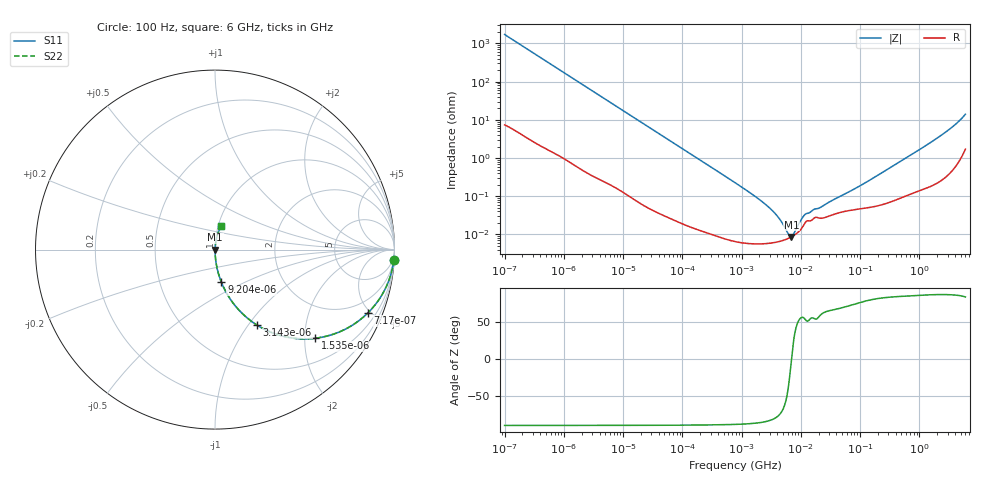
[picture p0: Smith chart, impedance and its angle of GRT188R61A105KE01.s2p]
!Murata Part Number: GRT188R61A105KE01
!These Parameters are Measured in Series Mode Connection
!Data Generated on Jun 19, 2026
!  o--ll--o
!Port1  Port2
!  o------o
!Operation Temp=25[degC], DC Bias Voltage=0[V]
!Freq. Start=100[Hz] Stop=6[GHz] 401[Steps]
# Hz S RI R 50
!Freq.(Hz) S11(Real) S11(Imag) S21(Real) S21(Imag) S12(Real) S12(Imag) S22(Real) S22(Imag)
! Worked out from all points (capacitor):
!   401 points, 100 Hz to 6 GHz, reference 50 ohm
!   read as one part in series: C = 928 nF near 109 Hz
!   lowest |Z| = 8.66 mohm at 6.949 MHz (marker M1)
!   series resonance near 6.96 MHz, so ESL is about 560 pH
!   S11 on the Smith chart (normalised r, x): 100 Hz: 1, -34; 717 Hz: 1.03, -4.81; 1.535 kHz: 1.01, -2.25; 3.143 kHz: 1.01, -1.10; 9.204 kHz: 1.00, -0.38; 6 GHz: 1.03, +0.28
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100  0.9964 -0.0582  0.00364 0.0582  0.00364 0.0582  0.9964 -0.0582
335  0.9626 -0.1874  0.0374 0.1874  0.0374 0.1874  0.9626 -0.1874
717  0.8511 -0.3533  0.1489 0.3533  0.1489 0.3533  0.8511 -0.3533
1535  0.5587 -0.4937  0.4413 0.4937  0.4413 0.4937  0.5587 -0.4937
2008  0.4264 -0.4917  0.5736 0.4917  0.5736 0.4917  0.4264 -0.4917
3143  0.2345 -0.4207  0.7655 0.4207  0.7655 0.4207  0.2345 -0.4207
5143  0.1039 -0.3018  0.8961 0.3018  0.8961 0.3018  0.1039 -0.3018
9204  0.0358 -0.1821  0.9642 0.1821  0.9642 0.1821  0.0358 -0.1821
40335  0.00224 -0.0433  0.9978 0.0433  0.9978 0.0433  0.00224 -0.0433
774597  7.03e-05 -0.00227  0.9999 0.00227  0.9999 0.00227  7.03e-05 -0.00227
1734173  5.76e-05 -0.000965  0.9999 0.000965  0.9999 0.000965  5.76e-05 -0.000965
2967816  5.91e-05 -0.000491  0.9999 0.000491  0.9999 0.000491  5.91e-05 -0.000491
4246196  6.49e-05 -0.000264  0.9999 0.000264  0.9999 0.000264  6.49e-05 -0.000264
6075234  7.82e-05 -6.99e-05  0.9999 6.99e-05  0.9999 6.99e-05  7.82e-05 -6.99e-05
6948629  8.66e-05 -8e-07  0.9999 8e-07  0.9999 8e-07  8.66e-05 -8e-07
7947587  9.83e-05 6.86e-05  0.9999 -6.86e-05  0.9999 -6.86e-05  9.83e-05 6.86e-05
1.137099e7  0.000183 0.000257  0.9998 -0.000257  0.9998 -0.000257  0.000183 0.000257
1.555665e7  0.000241 0.000345  0.9998 -0.000345  0.9998 -0.000345  0.000241 0.000345
8.527865e7  0.000453 0.00157  0.9995 -0.00157  0.9995 -0.00157  0.000453 0.00157
3.124326e8  0.000718 0.00538  0.9993 -0.00538  0.9993 -0.00538  0.000718 0.00538
2.240541e9  0.00383 0.0372  0.9962 -0.0372  0.9962 -0.0372  0.00383 0.0372
6e9  0.0349 0.1322  0.9651 -0.1322  0.9651 -0.1322  0.0349 0.1322
